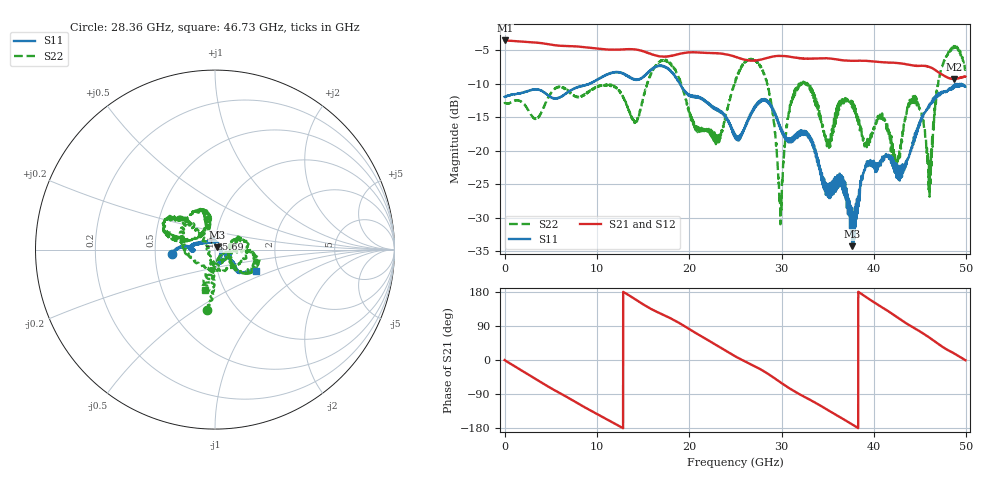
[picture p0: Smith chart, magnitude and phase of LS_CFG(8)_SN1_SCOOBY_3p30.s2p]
!Keysight Technologies,N5245B,MY58422026,A.13.80.08
!Date: Thursday, March 19, 2020 23:29:09
!Correction: S11(Full 2 Port(1,2))
!S21(Full 2 Port(1,2))
!S12(Full 2 Port(1,2))
!S22(Full 2 Port(1,2))
!S2P File: Measurements: S11, S21, S12, S22:
# Hz S DB R 50.0
!freq dBS11 angS11 dBS21 angS21 dBS12 angS12 dBS22 angS22
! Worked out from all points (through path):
!   4991 points, 10 MHz to 49.91 GHz, reference 50 ohm
!   highest |S21| = -3.56 dB at 20 MHz (marker M1); lowest = -9.3 dB at 48.67 GHz (marker M2)
!   group delay of S21, straight-line fit = 39.7 ps
!   lowest |S11| = -34.3 dB at 37.65 GHz (marker M3), VSWR 1.04, Z = 51.4 + j1.39 ohm
!   |S11| at or under -10 dB: start of sweep to 9.206 GHz; 9.257154 GHz to 9.28704 GHz (29.89 MHz wide, 0.322 % of centre); 18.98 GHz to end of sweep
!   |S22| runs from -31.0 to -4.4 dB; largest |S21 - S12| = 0.0061
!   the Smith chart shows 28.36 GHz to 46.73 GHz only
!   S11 on the Smith chart (normalised r, x): 28.36 GHz: 0.61, -0.03; 35.69 GHz: 0.95, +0.11; 46.73 GHz: 1.53, -0.38
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1e7  -11.97 -0.9  -3.56 -0.3  -3.55 -0.3  -12.75 0.1
2e7  -11.95 -0.5  -3.56 -0.4  -3.55 -0.4  -12.84 -0.5
4.24e9  -11.29 -54.1  -4.01 -63.0  -4.00 -63.0  -13.53 -80.0
8.33e9  -10.43 -80.7  -4.52 -119.8  -4.51 -119.8  -11.90 -93.3
1.419e10  -9.44 -128.0  -4.91 159.7  -4.91 159.8  -15.78 -139.3
1.665e10  -7.37 -138.4  -5.89 125.3  -5.88 125.3  -6.90 -166.8
2.299e10  -14.01 -169.2  -5.46 38.7  -5.46 38.8  -18.58 -154.4
2.496e10  -17.79 -163.7  -5.97 10.1  -5.96 10.2  -9.79 -168.5
2.836e10  -12.40 -173.7  -6.21 -33.8  -6.21 -33.7  -9.45 -97.7
2.988e10  -16.79 172.7  -5.88 -59.0  -5.87 -58.8  -31.00 -166.6
3.115e10  -18.14 -175.7  -6.05 -79.0  -6.05 -78.8  -12.04 138.2
3.328e10  -18.39 163.0  -6.27 -107.8  -6.27 -107.5  -11.12 163.9
3.569e10  -24.19 111.8  -6.34 -141.7  -6.28 -141.4  -15.13 102.3
3.765e10  -34.27 44.5  -6.59 -169.6  -6.52 -169.8  -13.02 139.5
3.917e10  -22.35 -75.1  -6.61 165.8  -6.59 165.6  -18.77 -107.5
4.16e10  -20.82 -10.1  -6.88 128.1  -6.90 127.9  -17.57 27.5
4.253e10  -22.47 -15.1  -6.93 113.1  -6.95 113.0  -22.00 -13.0
4.445e10  -17.43 -36.8  -7.31 82.8  -7.33 82.9  -12.19 -17.4
4.603e10  -13.14 -36.8  -7.52 58.7  -7.54 58.7  -26.89 -45.8
4.673e10  -11.84 -27.2  -8.06 46.7  -8.08 46.8  -12.68 -103.8
4.867e10  -10.23 -49.4  -9.31 17.5  -9.33 17.6  -4.44 -59.5
4.991e10  -10.49 -45.0  -8.94 -0.6  -8.96 -0.8  -7.91 -27.7
